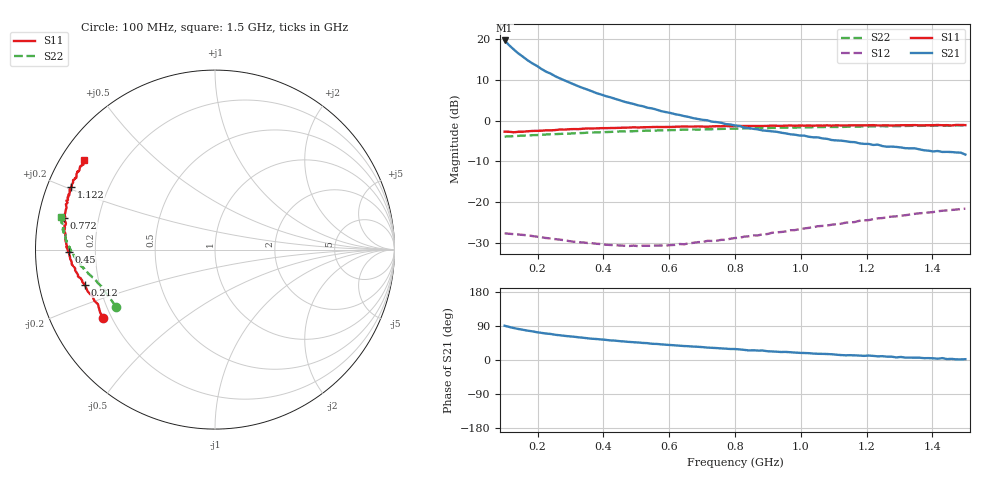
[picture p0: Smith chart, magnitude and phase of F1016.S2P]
!  POLYFET RF DEVICES
!  S PARAMETERS FOR
!  F1016 (Each Side)
!  VDS=28, IDQ=200mA
! Date: Mon Oct 21 17:40:39 1991
! Bias (V mA) : V1=2.3989000  I1=0.0047421  V2=27.998800  I2=208.57320
# MHZ S MA R 50
!  FREQ  S11 MAG  S11 ANG  S21 MAG  S21 ANG  S12 MAG  S12 ANG S22 MAG  S22 ANG
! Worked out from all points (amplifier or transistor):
!   101 points, 100 MHz to 1.5 GHz, reference 50 ohm
!   highest |S21| = 19.7 dB at 100 MHz (marker M1)
!   |S21| within 3 dB of that: start of sweep to 139.2 MHz
!   unconditionally stable (mu >= 1): 404.3 MHz to 1.408 GHz; 1.423 GHz to 1.437 GHz; 1.453 GHz to 1.46 GHz
!   at 324 MHz: K = 0.77, MSG = 19.1 dB, |S12| = -29.8 dB
!   at 800 MHz: K = 1.48, MAG = 9.7 dB, |S12| = -28.8 dB
!   at 1.5 GHz: K = 0.99, MSG = 6.6 dB, |S12| = -21.6 dB
!   S11 on the Smith chart (normalised r, x): 100 MHz: 0.17, -0.27; 212 MHz: 0.14, -0.13; 450 MHz: 0.10, -0.01; 772 MHz: 0.08, +0.10; 1.122 GHz: 0.07, +0.21; 1.5 GHz: 0.07, +0.31
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100  0.7319 -148.6  9.625 90.4  0.04151 8.0  0.6373 -150.2
114  0.7294 -151.4  8.393 87.3  0.04092 5.8  0.6407 -153.1
128  0.7196 -155.0  7.454 84.3  0.04053 4.0  0.6455 -155.4
142  0.73 -157.0  6.661 81.8  0.04012 3.1  0.6499 -157.1
170  0.74 -160.6  5.493 77.5  0.03919 1.0  0.6557 -159.9
184  0.747 -161.9  5.048 75.6  0.03839 1.2  0.6632 -160.8
198  0.7488 -163.3  4.691 73.4  0.0377 0.6  0.6649 -162.1
212  0.7519 -165.0  4.302 71.6  0.03708 0.8  0.6707 -163.0
226  0.761 -166.3  3.986 69.9  0.03629 0.5  0.6757 -163.6
268  0.7779 -168.9  3.296 65.2  0.03464 1.2  0.6871 -165.6
296  0.7836 -170.9  2.949 62.5  0.03326 1.9  0.6929 -166.8
338  0.7951 -173.4  2.513 58.8  0.03202 4.6  0.7052 -168.1
380  0.8033 -175.6  2.167 55.3  0.03082 6.7  0.7181 -169.2
450  0.8155 -179.1  1.778 49.7  0.02938 12.0  0.736 -171.1
576  0.8341 175.7  1.307 41.3  0.02941 25.1  0.7613 -174.2
674  0.8449 171.6  1.07 35.4  0.03171 34.3  0.7784 -176.5
772  0.8591 168.3  0.9067 30.0  0.03447 41.9  0.7939 -178.1
800  0.8579 167.3  0.8731 29.0  0.03632 43.5  0.7953 -179.0
1038  0.8667 159.5  0.6244 17.0  0.04929 52.7  0.8316 176.5
1122  0.8721 156.5  0.5682 13.0  0.0543 54.1  0.8359 174.5
1276  0.8702 152.5  0.4802 8.8  0.06641 55.0  0.8552 172.1
1500  0.881 145.7  0.3831 2.1  0.08332 53.2  0.8761 168.0
